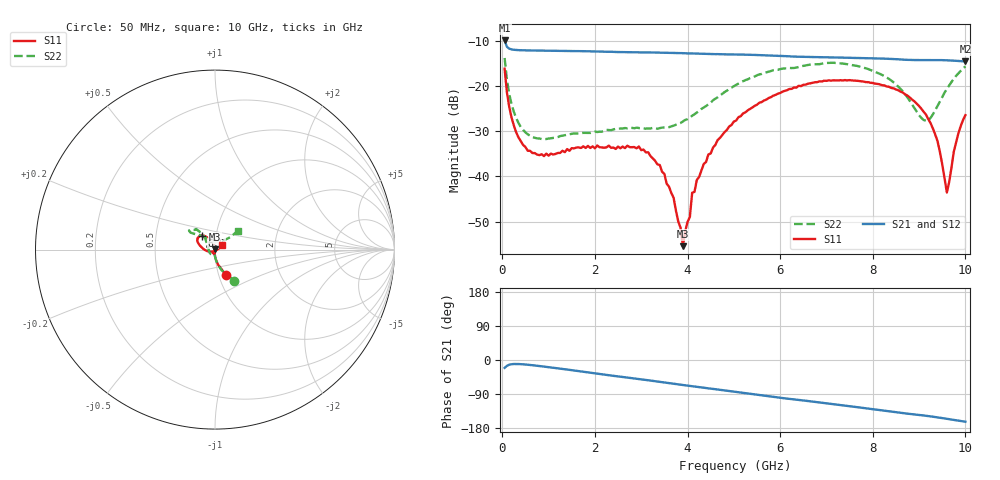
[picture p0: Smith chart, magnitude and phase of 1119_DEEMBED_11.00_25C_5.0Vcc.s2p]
!Hittite Microwave Corp.
!Digital Attenuator/PhaseShifter Rev 1.4.0
!Filename: C:\DATA\DATA\1119_DEEMBED_11.00_25C_5.0Vcc.s2p
!VNA ID: Agilent Technologies,N5224A,MY51441122,A.10.45.03
!Device type:
!2 Port Calibration.
!Temp(C): 25
!Lot Number:
!Serial Number:
!Operator:
!Misc:
!Attenuator:  11.000
# GHZ S DB R 50.0
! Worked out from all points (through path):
!   200 points, 50 MHz to 10 GHz, reference 50 ohm
!   highest |S21| = -9.96 dB at 50 MHz (marker M1); lowest = -14.6 dB at 10 GHz (marker M2)
!   group delay of S21, straight-line fit = 43.5 ps
!   lowest |S11| = -55.4 dB at 3.9 GHz (marker M3), VSWR 1.00, Z = 49.8 + j0.0594 ohm
!   |S11| at or under -10 dB: start of sweep to end of sweep
!   |S22| runs from -31.8 to -13.8 dB; largest |S21 - S12| = 0.00081
!   S11 on the Smith chart (normalised r, x): 50 MHz: 1.08, -0.32; 6.6 GHz: 0.86, +0.13; 10 GHz: 1.08, +0.06
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0.05  -16.20 -66.7  -9.96 -20.9  -9.96 -20.9  -13.83 -58.2
0.1  -21.44 -78.7  -11.37 -15.5  -11.36 -15.5  -18.62 -73.1
0.2  -27.02 -87.2  -11.93 -11.2  -11.94 -11.2  -24.06 -83.8
0.55  -34.35 -99.0  -12.16 -12.5  -12.16 -12.5  -30.71 -94.5
1.75  -33.36 -115.4  -12.33 -30.9  -12.34 -31.0  -30.38 -111.4
2.95  -33.40 -106.1  -12.59 -50.2  -12.60 -50.3  -29.32 -148.7
3.4  -37.49 -111.0  -12.65 -57.6  -12.65 -57.7  -29.33 -169.8
3.7  -44.75 -115.0  -12.71 -62.7  -12.72 -62.8  -28.79 174.1
3.9  -55.43 159.4  -12.77 -66.1  -12.78 -66.1  -27.87 163.3
4.05  -48.99 113.5  -12.82 -68.4  -12.83 -68.5  -27.00 154.8
4.1  -43.62 108.7  -12.83 -69.3  -12.84 -69.3  -26.60 152.6
4.2  -40.82 101.9  -12.88 -70.9  -12.89 -71.0  -25.88 147.5
4.65  -31.98 100.7  -12.98 -77.9  -13.01 -77.9  -22.52 133.8
5.05  -27.66 108.5  -13.07 -84.1  -13.08 -84.2  -19.78 129.2
6.6  -19.52 132.9  -13.60 -108.2  -13.61 -108.3  -15.38 139.6
6.7  -19.31 134.5  -13.61 -109.8  -13.62 -109.8  -15.24 140.1
8.35  -20.20 160.1  -14.03 -135.5  -14.03 -135.5  -18.46 137.1
9.15  -26.37 -171.6  -14.29 -147.2  -14.30 -147.2  -27.72 87.6
9.400001  -32.29 -151.3  -14.29 -151.4  -14.30 -151.4  -24.41 52.3
9.6  -43.57 -74.5  -14.35 -155.2  -14.36 -155.2  -20.67 41.4
9.75  -34.54 12.7  -14.43 -158.1  -14.44 -158.1  -18.42 39.1
10  -26.46 36.4  -14.61 -162.9  -14.61 -162.9  -15.70 39.9
